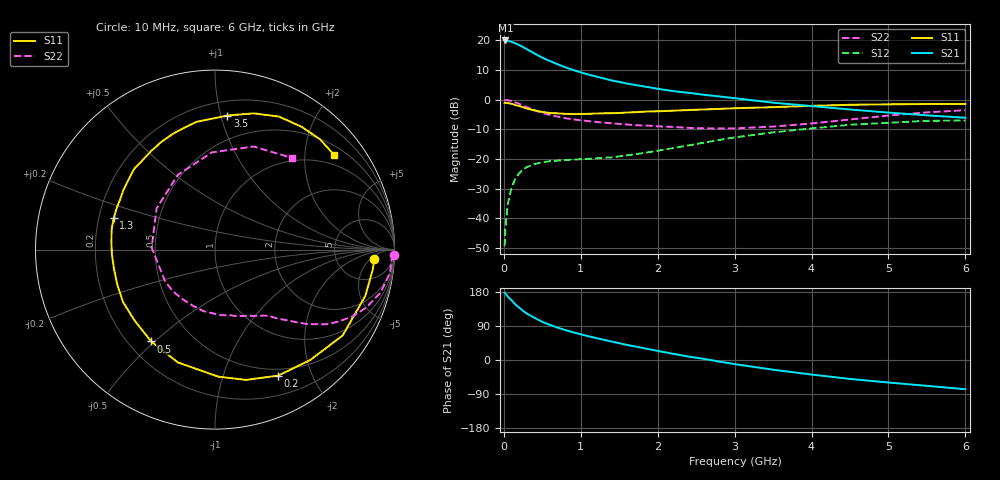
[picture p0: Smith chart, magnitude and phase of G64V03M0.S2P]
! SIEMENS Small Signal Semiconductors
! BFG193
! Si NPN RF Bipolar Junction Transistor in SOT223
! VCE = 4 V  IC = 3 mA
! Common Emitter S-Parameters:  August  1996
# GHz  S  MA  R  50
!  f  S11  S21  S12  S22
! GHz  MAG  ANG  MAG  ANG  MAG  ANG  MAG  ANG
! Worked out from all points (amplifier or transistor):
!   36 points, 10 MHz to 6 GHz, reference 50 ohm
!   highest |S21| = 20.0 dB at 20 MHz (marker M1)
!   |S21| within 3 dB of that: start of sweep to 302.8 MHz
!   unconditionally stable (mu >= 1): 1.282 GHz to 2.539 GHz
!   at 250 MHz: K = 0.23, MSG = 20.6 dB, |S12| = -23.5 dB
!   at 1.4 GHz: K = 1.08, MAG = 11.3 dB, |S12| = -19.4 dB
!   at 6 GHz: K = 0.91, MSG = 0.5 dB, |S12| = -7.0 dB
!   S11 on the Smith chart (normalised r, x): 10 MHz: 13, -7; 200 MHz: 0.42, -1.54; 500 MHz: 0.29, -0.49; 1.3 GHz: 0.26, +0.14; 3.5 GHz: 0.31, +1.05; 6 GHz: 0.72, +2.70
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0.01  0.8887 -3.5  9.931 177.5  0.0034 90.4  0.9951 -1.6
0.02  0.8861 -7.1  9.998 176.0  0.0067 90.4  0.9859 -3.0
0.05  0.8766 -17.1  9.879 167.6  0.0172 79.4  0.9838 -7.5
0.1  0.8573 -33.9  9.487 157.9  0.0329 72.9  0.9535 -14.5
0.15  0.8124 -49.3  8.923 146.4  0.047 63.4  0.9026 -20.9
0.2  0.7852 -63.4  8.344 138.1  0.0577 57.7  0.8531 -25.8
0.25  0.7463 -76.6  7.729 129.6  0.067 51.5  0.7971 -30.2
0.3  0.7082 -88.5  7.111 122.4  0.0733 47.3  0.7499 -33.7
0.4  0.6618 -108.2  6.02 111.1  0.0826 39.8  0.6627 -38.8
0.5  0.6231 -124.8  5.114 100.7  0.0881 34.6  0.5998 -42.2
0.6  0.5977 -138.4  4.494 92.6  0.0923 31.6  0.5548 -45.0
0.7  0.59 -150.3  3.976 85.4  0.0941 29.5  0.5186 -47.8
0.9  0.573 -169.1  3.178 73.1  0.0983 27.8  0.4669 -52.1
1.1  0.5791 175.7  2.655 62.7  0.1009 27.8  0.4361 -57.9
1.3  0.5907 162.8  2.287 53.3  0.1055 29.3  0.411 -63.5
1.6  0.6093 146.8  1.874 39.7  0.1156 31.8  0.3834 -74.3
2.2  0.6542 123.0  1.4 16.4  0.1534 33.7  0.3487 -100.7
2.8  0.702 103.6  1.137 -4.1  0.2102 28.3  0.3303 -134.9
3.5  0.7502 84.7  0.893 -25.6  0.2818 14.0  0.3531 178.2
4.5  0.8227 64.2  0.685 -50.0  0.3785 -8.3  0.465 116.4
5.5  0.8484 46.5  0.546 -68.2  0.4419 -36.1  0.6133 69.5
6  0.8479 38.4  0.497 -77.1  0.4462 -51.4  0.6667 50.0
